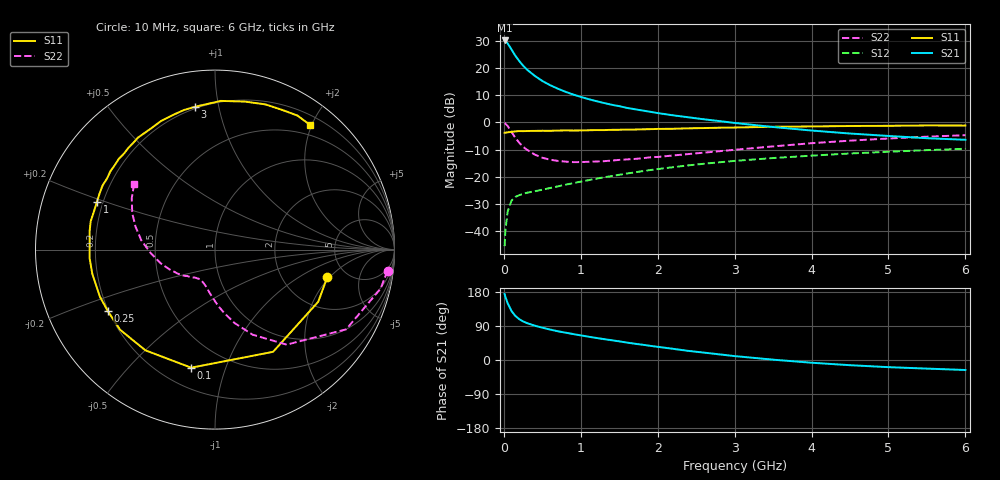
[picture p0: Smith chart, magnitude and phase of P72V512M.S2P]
! SIEMENS Small Signal Semiconductors
! BFP196
! Si NPN RF Bipolar Junction Transistor in SOT143
! VCE = 2.5 V  IC = 12 mA
! Common Emitter S-Parameters:  May  1996
# GHz  S  MA  R  50
!  f  S11  S21  S12  S22
! GHz  MAG  ANG  MAG  ANG  MAG  ANG  MAG  ANG
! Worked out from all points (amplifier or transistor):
!   36 points, 10 MHz to 6 GHz, reference 50 ohm
!   highest |S21| = 30.1 dB at 10 MHz (marker M1)
!   |S21| within 3 dB of that: start of sweep to 92.43 MHz
!   unconditionally stable (mu >= 1): 831.4 MHz to 3.384 GHz
!   at 250 MHz: K = 0.46, MSG = 23.5 dB, |S12| = -26.3 dB
!   at 1.4 GHz: K = 1.13, MAG = 10.9 dB, |S12| = -19.8 dB
!   at 6 GHz: K = 0.97, MSG = 1.7 dB, |S12| = -9.7 dB
!   S11 on the Smith chart (normalised r, x): 10 MHz: 3.59, -1.87; 100 MHz: 0.32, -0.77; 250 MHz: 0.20, -0.26; 1 GHz: 0.18, +0.19; 3 GHz: 0.19, +0.85; 6 GHz: 0.33, +1.96
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0.01  0.6446 -13.7  31.98 174.2  0.0053 84.4  0.969 -7.0
0.02  0.6444 -26.8  31.05 166.7  0.0103 78.7  0.9475 -13.3
0.05  0.655 -60.4  28.16 149.8  0.0232 64.2  0.8552 -31.3
0.1  0.6712 -101.4  21.78 129.2  0.0364 48.5  0.6631 -53.0
0.15  0.682 -124.6  16.72 116.2  0.0427 40.6  0.5188 -66.1
0.2  0.6921 -139.8  13.43 107.8  0.0459 36.9  0.4222 -75.2
0.25  0.6884 -150.1  11.01 101.8  0.0486 35.0  0.3553 -81.9
0.3  0.6929 -157.8  9.348 97.4  0.0508 35.0  0.3142 -86.8
0.4  0.6968 -168.8  7.176 90.7  0.0541 35.1  0.256 -94.8
0.5  0.7005 -176.3  5.763 85.3  0.0577 37.2  0.2236 -100.9
0.6  0.6986 177.5  4.83 80.4  0.062 39.0  0.2059 -105.5
0.7  0.7059 171.6  4.17 75.9  0.0665 40.8  0.1957 -109.4
0.8  0.7104 167.2  3.653 72.2  0.0713 41.9  0.1898 -113.2
1  0.7093 158.0  2.935 65.0  0.0814 44.4  0.1861 -119.0
1.1  0.7151 154.1  2.675 61.5  0.0865 45.2  0.1883 -121.6
1.6  0.7365 136.8  1.844 46.0  0.1147 45.9  0.2083 -133.4
2.2  0.7618 118.8  1.346 29.5  0.15 42.7  0.246 -146.7
3  0.8034 98.0  0.975 10.3  0.1956 35.0  0.3131 -166.1
3.5  0.829 87.8  0.821 0.9  0.2208 29.5  0.3615 -177.4
4.5  0.8563 70.9  0.623 -13.7  0.2677 18.5  0.4608 163.9
5.5  0.8769 58.4  0.511 -22.7  0.3087 7.3  0.545 148.3
6  0.8736 52.9  0.478 -26.4  0.3268 1.2  0.5804 141.0
